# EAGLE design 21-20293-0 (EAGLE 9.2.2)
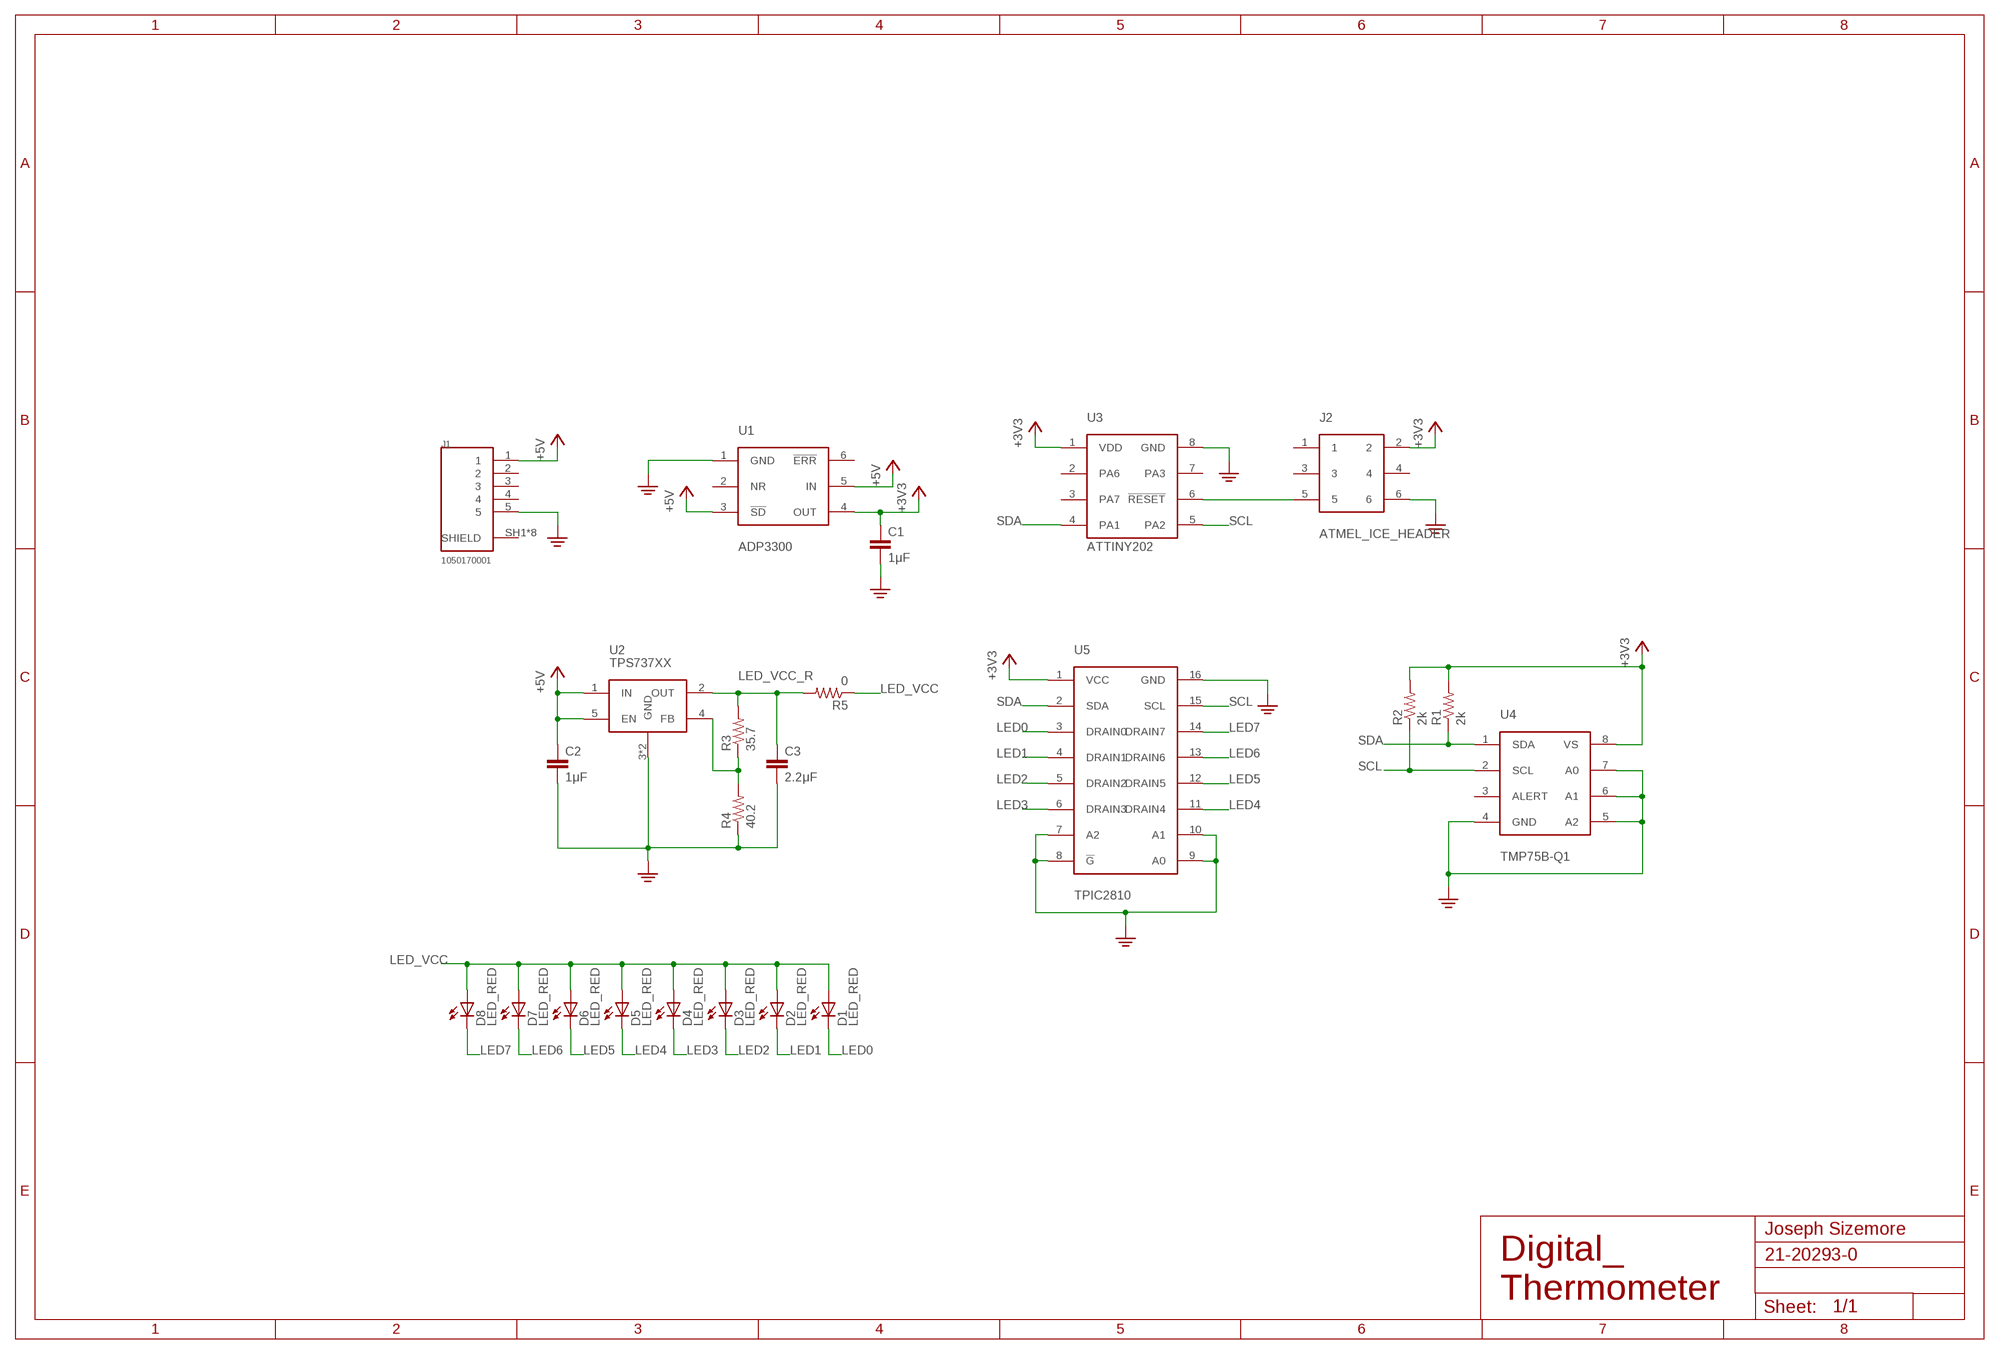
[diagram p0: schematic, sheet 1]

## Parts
C1  1μF  C-EUC0603  [C0603]
C2  1μF  C-EUC0603  [C0603]
C3  2.2μF  C-EUC0603  [C0603]
D1  LED_RED  [STANDARD_RED_LED]
D2  LED_RED  [STANDARD_RED_LED]
D3  LED_RED  [STANDARD_RED_LED]
D4  LED_RED  [STANDARD_RED_LED]
D5  LED_RED  [STANDARD_RED_LED]
D6  LED_RED  [STANDARD_RED_LED]
D7  LED_RED  [STANDARD_RED_LED]
D8  LED_RED  [STANDARD_RED_LED]
J1  1050170001  [MOLEX_1050170001]
J2  ATMEL_ICE_HEADER  [ATMEL_ICE_HEADER]
R1  2k  R-US_R0603  [R0603]
R2  2k  R-US_R0603  [R0603]
R3  35.7  R-US_R0603  [R0603]
R4  40.2  R-US_R0603  [R0603]
R5  0  R-US_R0603  [R0603]
U1  ADP3300  [8-PIN_SOT-23]
U2  TPS737XX  [SOT-223]
U3  ATTINY202  [8-PIN_SOIC150]
U4  TMP75B-Q1  [8-PIN_SOIC150]
U5  TPIC2810  [16-PIN_SOIC150]

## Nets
+3V3: C1.1 J2.2 R1.2 R2.2 U1.4(OUT) U3.1(VDD) U4.8(VS) U5.1(VCC)
+5V: C2.1 J1.1 U1.3(!SD!) U1.5(IN) U2.1(IN) U2.5(EN)
GND: C1.2 C2.2 C3.2 J1.5 J2.6 R4.1 U1.1(GND) U2.3(GND) U2.6(GND) U3.8(GND) U4.4(GND) U4.5(A2) U4.6(A1) U4.7(A0) U5.7(A2) U5.8(!G!) U5.9(A0) U5.10(A1) U5.16(GND) ; supply symbol labelled PE
LED0: D1.CATHODE U5.3(DRAIN0)
LED1: D2.CATHODE U5.4(DRAIN1)
LED2: D3.CATHODE U5.5(DRAIN2)
LED3: D4.CATHODE U5.6(DRAIN3)
LED4: D5.CATHODE U5.11(DRAIN4)
LED5: D6.CATHODE U5.12(DRAIN5)
LED6: D7.CATHODE U5.13(DRAIN6)
LED7: D8.CATHODE U5.14(DRAIN7)
LED_VCC: D1.ANODE D2.ANODE D3.ANODE D4.ANODE D5.ANODE D6.ANODE D7.ANODE D8.ANODE R5.1
LED_VCC_FB: R3.1 R4.2 U2.4(FB)
LED_VCC_R: C3.1 R3.2 R5.2 U2.2(OUT)
N$1: J2.5 U3.6(!RESET!)
SCL: R2.1 U3.5(PA2) U4.2(SCL) U5.15(SCL)
SDA: R1.1 U3.4(PA1) U4.1(SDA) U5.2(SDA)
Unconnected: J1.2 J1.3 J1.4 J1.SH1(SHIELD) J1.SH2(SHIELD) J1.SH3(SHIELD) J1.SH4(SHIELD) J1.SH5(SHIELD) J1.SH6(SHIELD) J1.SH7(SHIELD) J1.SH8(SHIELD) J2.1 J2.3 J2.4 U1.2(NR) U1.6(!ERR!) U3.2(PA6) U3.3(PA7) U3.7(PA3) U4.3(ALERT)

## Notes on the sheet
- Joseph Sizemore
- Digital_
  Thermometer

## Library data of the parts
C1-C3 = rcl:C-EU: CAPACITOR, European symbol; SPICEPREFIX: C
D1-D8 = Diodes:LED_RED
J1 = 1050170001:1050170001: Conn.; Data; USB; Recept.; Micro; B Type; Bottom Mount, SMT, with Solder Tabs, Lead-Free; DESCRIPTION: Conn.; Data; USB; Recept.; Micro; B Type; Bottom Mount, SMT, with Solder Tabs, Lead-Free; DIGI-KEY_PART_NUMBER: WM1399CT-ND; DIGI-KEY_PURCHASE_URL: https://www.digikey.com/product-detail/en/molex/1050170001/WM1399CT-ND/2350885?utm_source=snapeda&utm_medium=aggregator&utm_campaign=symbol; MF: Molex; MP: 1050170001; PACKAGE: None
J2 = Headers:ATMEL_ICE_HEADER
R1-R5 = rcl:R-US_: RESISTOR, American symbol; SPICEPREFIX: R
U1 = Linear Regulators:ADP3300
U2 = Linear Regulators:TPS737XX
U3 = Microcontrollers:ATTINY202
U4 = Peripherals:TMP75B-Q1
U5 = Peripherals:TPIC2810

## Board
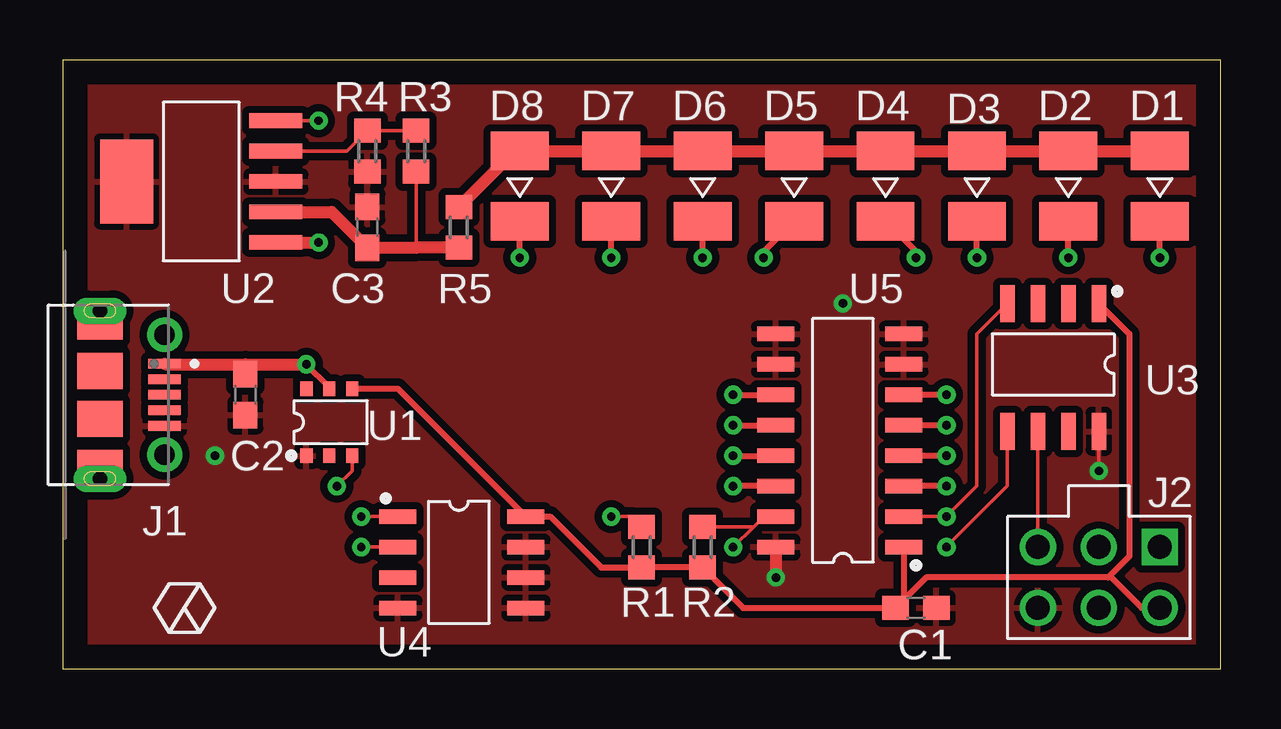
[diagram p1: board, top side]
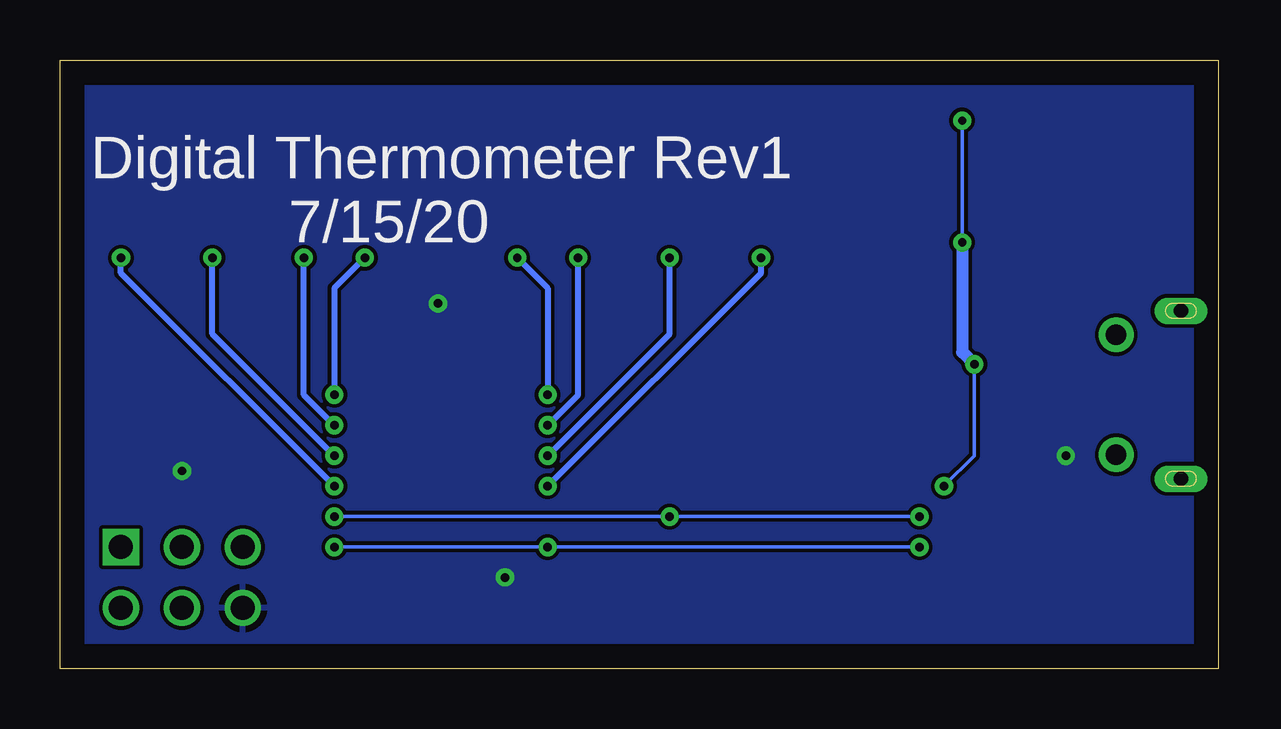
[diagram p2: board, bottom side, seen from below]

Size 48.26 x 25.39 mm. Coordinates in mm from the lower left corner, seen from the top.
Outline: 0,0 48.26,0 48.26,25.39 0,25.39 0,0
Copper layers (1*16): Top 0.035mm / dielectric 1.5mm / Bottom 0.035mm
Design rules "default": minimum track width 6mil, minimum drill 0.35mm, track to track 6mil, track to pad 6mil, pad to pad 6mil, via to via 6mil, smd to smd 6mil, copper to edge 40mil, drill to drill 6mil, minimum pad ring 10mil, minimum via ring 8mil, stop-mask expansion 4mil, vias tented up to drill 0mil, thermal gap 10mil

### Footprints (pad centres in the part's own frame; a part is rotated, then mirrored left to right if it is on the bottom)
C0603 = smd 1.1 x 1: 1 -0.85,0; 2 0.85,0
STANDARD_RED_LED = smd 1.6 x 2.413: ANODE 0,0; CATHODE 2.921,0
MOLEX_1050170001 = smd 0.4 x 1.35: 1 -1.3,2.35; 2 -0.65,2.35; 3 0,2.35; 4 0.65,2.35; 5 1.3,2.35 | drill 0.85 pad 1.45: SH1 -2.5,2.35; SH2 2.5,2.35 | drill 0.6 pad 0.95 long: SH3 -3.5,-0.35; SH8 3.5,-0.35 | smd 1.2 x 1.9: SH4 -2.9,-0.35; SH7 2.9,-0.35 | smd 1.5 x 1.9: SH5 -1,-0.35; SH6 1,-0.35
ATMEL_ICE_HEADER = drill 1 square: 1 0,0 | drill 1: 2 2.54,0; 3 0,-2.54; 4 2.54,-2.54; 5 0,-5.08; 6 2.54,-5.08
R0603 = smd 1 x 1.1: 1 -0.85,0; 2 0.85,0
8-PIN_SOT-23 = smd 0.61 x 0.508: 1 0,0; 2 0,-0.953; 3 0,-1.905; 4 2.794,-1.905; 5 2.794,-0.953; 6 2.794,0
SOT-223 = smd 2.21 x 0.61: 1 0,0; 2 0,-1.27; 3 0,-2.54; 4 0,-3.81; 5 0,-5.08 | smd 2.21 x 3.505: 6 6.223,-2.54
8-PIN_SOIC150 = smd 1.549 x 0.61: 1 0,0; 2 0,-1.27; 3 0,-2.54; 4 0,-3.81; 5 5.334,-3.81; 6 5.334,-2.54; 7 5.334,-1.27; 8 5.334,0
16-PIN_SOIC150 = smd 1.549 x 0.61: 1 0,0; 2 0,-1.27; 3 0,-2.54; 4 0,-3.81; 5 0,-5.08; 6 0,-6.35; 7 0,-7.62; 8 0,-8.89; 9 5.334,-8.89; 10 5.334,-7.62; 11 5.334,-6.35; 12 5.334,-5.08; 13 5.334,-3.81; 14 5.334,-2.54; 15 5.334,-1.27; 16 5.334,0

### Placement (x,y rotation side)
C1  35.56,2.54 0 top
C2  7.62,11.43 270 top
C3  12.7,18.41 90 top
D1  45.72,21.59 270 top
D2  41.91,21.59 270 top
D3  38.1,21.59 270 top
D4  34.29,21.59 270 top
D5  30.48,21.59 270 top
D6  26.67,21.59 270 top
D7  22.86,21.59 270 top
D8  19.05,21.59 270 top
J1  1.91,11.43 270 top
J2  45.72,5.08 270 top
R1  24.13,5.08 270 top
R2  26.67,5.08 270 top
R3  14.73,21.59 270 top
R4  12.7,21.59 90 top
R5  16.51,18.41 270 top
U1  10.16,8.89 90 top
U2  8.89,17.78 180 top
U3  43.18,15.24 270 top
U4  13.97,6.35 0 top
U5  35.05,5.08 180 top

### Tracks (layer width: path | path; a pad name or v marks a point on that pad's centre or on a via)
+3V3
  Top 0.152: 35.05,2.88 C1.1
  Top 0.254: U1.4 13.97,11.68 U4.8 20.32,6.35 22.44,4.23 R1.2 R2.2 28.36,2.54 C1.1 | U3.1 44.45,13.97 44.45,4.7 43.62,3.87 | U5.1 35.05,2.88 35.98,3.81 43.56,3.81 43.62,3.87 | J2.2 44.96,2.54 43.62,3.87
+5V  (via drill 0.35)
  Top 0.152: v10.67,22.86 U2.5 | U1.5 11.11,11.75 | v11.43,7.62 12.06,8.26 U1.3 | C2.1 7.62,12.7
  Top 0.254: 11.11,11.75 v10.16,12.7
  Top 0.508: U2.1 v10.67,17.78 | J1.1 4.29,12.7 7.62,12.7 v10.16,12.7
  Bottom 0.152: v10.67,22.86 v10.67,17.78 | v10.16,12.7 10.16,8.89 v11.43,7.62
  Bottom 0.508: v10.67,17.78 10.67,13.21 v10.16,12.7
GND  (via drill 0.35)
  Top 0.152: U3.8 v43.18,8.26
  Top 0.508: U5.16 v29.72,3.81
  other vias: 6.35,8.89 32.51,15.24
  pour Top (isolate 0.305): 0,0 48.26,0 48.26,25.4 0,25.4
  pour Bottom: 0,0 48.26,0 48.26,25.4 0,25.4
LED0  (via drill 0.35)
  Top 0.254: v45.72,17.14 D1.CATHODE | v36.83,7.62 U5.3
  Bottom 0.254: v36.83,7.62 45.72,16.51 v45.72,17.14
LED1  (via drill 0.35)
  Top 0.254: v41.91,17.14 D2.CATHODE | v36.83,8.89 U5.4
  Bottom 0.254: v36.83,8.89 41.91,13.97 v41.91,17.14
LED2  (via drill 0.35)
  Top 0.254: v38.1,17.14 D3.CATHODE | v36.83,10.16 U5.5
  Bottom 0.254: v36.83,10.16 38.1,11.43 v38.1,17.14
LED3  (via drill 0.35)
  Top 0.254: D4.CATHODE 35.56,17.4 v35.56,17.14 | v36.83,11.43 U5.6
  Bottom 0.254: v35.56,17.14 36.83,15.88 v36.83,11.43
LED4  (via drill 0.35)
  Top 0.254: D5.CATHODE 29.21,17.4 v29.21,17.14 | v27.94,11.43 U5.11
  Bottom 0.254: v29.21,17.14 27.94,15.88 v27.94,11.43
LED5  (via drill 0.35)
  Top 0.254: v26.67,17.14 D6.CATHODE | v27.94,10.16 U5.12
  Bottom 0.254: v27.94,10.16 26.67,11.43 v26.67,17.14
LED6  (via drill 0.35)
  Top 0.254: v22.86,17.14 D7.CATHODE | v27.94,8.89 U5.13
  Bottom 0.254: v27.94,8.89 22.86,13.97 v22.86,17.14
LED7  (via drill 0.35)
  Top 0.254: U5.14 v27.94,7.62 | v19.05,17.14 D8.CATHODE
  Bottom 0.254: v27.94,7.62 19.05,16.51 v19.05,17.14
LED_VCC
  Top 0.508: D1.ANODE D2.ANODE D3.ANODE D4.ANODE D5.ANODE D6.ANODE D7.ANODE D8.ANODE 18.84,21.59 R5.1
LED_VCC_FB
  Top 0.152: R3.1 R4.2 11.85,21.59 U2.4
LED_VCC_R
  Top 0.152: R3.2 14.73,17.57
  Top 0.508: U2.2 11.21,19.05 C3.1 14.73,17.57 R5.2
N$1
  Top 0.152: U3.6 J2.5
SCL  (via drill 0.35)
  Top 0.152: U5.15 29.21,6.35 28.79,5.93 | v27.94,5.08 28.79,5.93 | v36.83,5.08 39.37,7.62 U3.5 | R2.1 28.79,5.93 | U4.2 v12.45,5.08
  Bottom 0.152: v36.83,5.08 v27.94,5.08 v12.45,5.08
SDA  (via drill 0.35)
  Top 0.152: U3.4 38.1,13.97 38.1,7.62 v36.83,6.35 U5.2 | R1.1 23.71,6.35 v22.86,6.35 | U4.1 v12.45,6.35
  Bottom 0.152: v12.45,6.35 v22.86,6.35 v36.83,6.35

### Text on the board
bNames: Digital Thermometer Rev1 / 7/15/20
